FUNCTION_BLOCK "IMAC_STANDBY_CALL"
TITLE =Function calls for STANDBY objects
//*********************************************************************
//* Important : FB84 is only for use with FB80 (MOTOR1) !             *
//* STBY-Function for 2-speed or 2-direction drive is not available ! *
//*                                                                   *
//* Pumps 1 & 2 have to be allocated in different PLCs !              *
//* One PLC has the Standby Function AND one 'local' pump (MOTOR1)    *
//* The other PLCs has just one 'remote' pump (MOTOR1).               *
//* Both PLCs have to be linked by a Simatic data link to exchange    *
//* the Status & Command Words (ASTAT / ACOM) between STANDBY         *
//* function block and the 'remote' pump.                             *
//*********************************************************************
//
//Parameter Description for Function STANDBY (FB84):
//--------------------------------------------------
//OBJ:    Ascending Object number for STANDBY (1...x)
//
//C_O:    'CHANGE OVER' Input
//                      0 = Nothing to do
//                      1 = Change over command
//
//GSTA:   'GROUP START' Input
//                      0 = Nothing to do
//                      1 = Group Start (start one Motor, the other is in Standby)
//
//GSTO:   'GROUP STOP'  Input
//                      0 = Nothing to do
//                      1 = Group Start (start one Motor, the other is in Standby)
//
//FALT:   'EXT. FAULT'  Input
//                      0 = OK
//                      1 = Fault
//
//STAA:   'AUTO' Mode   Status Interface from MOTOR1 A
//                      Bit  8       : Running
//                      Bit  9       : Local
//                      Bit 10       : Manual
//                      Bit 11       : Auto
//                      Bit 12       : Failure
//                      Bit 13       : BlackOut
//                      Bit 14       : Starting
//                      Bit 15       : Restarting
//
//STAB:   'AUTO' Mode   Status Interface from MOTOR1 B (Bit assignment like STAA)
//
//PCONF:   (leave empty, refers to local instance data in Instance DB)
//
//ENAB:   'SPARE'       (not used)
//
//ACOA:   'AUTO' Mode   Command Interface to MOTOR1 A
//                      Bit  0       : BlackoutStart
//                      Bit  1       : StandbyActive
//                      Bit  7       : FetchData Command
//                      Bit  8       : Start Command
//                      Bit  9       : Stop  Command
//                      Bit 10       : Failure input from Automatic Function
//                      Bit 11       : Lock 'Start / Stop'
//                      Bit 12       : Emergency Off Command
//
//ACOB:   'AUTO' Mode   Command Interface to MOTOR1 B (Bit assignment like ACOA)
//
//OSSTAT:  OS Status Word (not used)
//
//OSALARM: OS Alarm Word  (not used)
//
//OSCOM:   OS Command Interface
//                      Bit  0       : Change Over  Command
//                      Bit  1       : Stop   Command
AUTHOR : HottendU
FAMILY : IMAC
VERSION : 0.2


VAR
  Standby_No001 : "IMAC_STANDBY";
  Standby_No002 : "IMAC_STANDBY";
  Standby_No003 : "IMAC_STANDBY";
  Standby_No004 : "IMAC_STANDBY";
  Standby_No005 : "IMAC_STANDBY";
  Standby_No006 : "IMAC_STANDBY";
  Standby_No007 : "IMAC_STANDBY";
  Standby_No008 : "IMAC_STANDBY";
  Standby_No009 : "IMAC_STANDBY";
  Standby_No010 : "IMAC_STANDBY";
END_VAR
BEGIN
NETWORK
TITLE =STANDBY Number 001

// Fetch 'ASTAT' Automatic Status Word' from first Pump ('local')
      L     "IMAC_MOTOR1_I/O".MOTOR1_005_ASTAT;
      T     "IMAC_STANDBY_I/O".STANDBY_001_STAA;

// Fetch 'ASTAT' Automatic Status Word'from Second Pump ('remote')
      L     "IMAC_MOTOR1_I/O".MOTOR1_006_ASTAT;
      T     "IMAC_STANDBY_I/O".STANDBY_001_STAB;

// Call Stanbdby Function
      CALL #Standby_No001 (
           OBJ                      := 1,
           C_O                      := E      9.2,
           GSTA                     := E      9.3,
           GSTO                     := E      9.4,
           FALT                     := E      9.5,
           STAA                     := "IMAC_STANDBY_I/O".STANDBY_001_STAA,
           STAB                     := "IMAC_STANDBY_I/O".STANDBY_001_STAB,
           ACOA                     := "IMAC_STANDBY_I/O".STANDBY_001_ACOA,
           ACOB                     := "IMAC_STANDBY_I/O".STANDBY_001_ACOB,
           OSSTAT                   := "IMAC_STANDBY_I/O".STANDBY_001_OSSTAT,
           OSALARM                  := "IMAC_STANDBY_I/O".STANDBY_001_OSALARM,
           OSCOM                    := "IMAC_STANDBY_I/O".STANDBY_001_OSCOM);

// Put 'ACOM' Automatic Command Word to first Pump (local')
      L     "IMAC_STANDBY_I/O".STANDBY_001_ACOA;
      T     "IMAC_MOTOR1_I/O".MOTOR1_005_ACOM;

// Put 'ACOM' Automatic Command Word to second Pump ('remote')
      L     "IMAC_STANDBY_I/O".STANDBY_001_ACOB;
      T     "IMAC_MOTOR1_I/O".MOTOR1_006_ACOM;
NETWORK
TITLE =STANDBY Number 002

//*********** END of function Processing ! *******************************************************************
      BEA   ; // Move this Instruction down to the next Network to add one object !
//************************************************************************************************************

      CALL #Standby_No002 (
           OBJ                      := 2,
           STAA                     := "IMAC_STANDBY_I/O".STANDBY_002_STAA,
           STAB                     := "IMAC_STANDBY_I/O".STANDBY_002_STAB,
           ACOA                     := "IMAC_STANDBY_I/O".STANDBY_002_ACOA,
           ACOB                     := "IMAC_STANDBY_I/O".STANDBY_002_ACOB,
           OSSTAT                   := "IMAC_STANDBY_I/O".STANDBY_002_OSSTAT,
           OSALARM                  := "IMAC_STANDBY_I/O".STANDBY_002_OSALARM,
           OSCOM                    := "IMAC_STANDBY_I/O".STANDBY_002_OSCOM);

NETWORK
TITLE =STANDBY Number 003

      CALL #Standby_No003 (
           OBJ                      := 3,
           STAA                     := "IMAC_STANDBY_I/O".STANDBY_003_STAA,
           STAB                     := "IMAC_STANDBY_I/O".STANDBY_003_STAB,
           ACOA                     := "IMAC_STANDBY_I/O".STANDBY_003_ACOA,
           ACOB                     := "IMAC_STANDBY_I/O".STANDBY_003_ACOB,
           OSSTAT                   := "IMAC_STANDBY_I/O".STANDBY_003_OSSTAT,
           OSALARM                  := "IMAC_STANDBY_I/O".STANDBY_003_OSALARM,
           OSCOM                    := "IMAC_STANDBY_I/O".STANDBY_003_OSCOM);

NETWORK
TITLE =STANDBY Number 004

      CALL #Standby_No004 (
           OBJ                      := 4,
           STAA                     := "IMAC_STANDBY_I/O".STANDBY_004_STAA,
           STAB                     := "IMAC_STANDBY_I/O".STANDBY_004_STAB,
           ACOA                     := "IMAC_STANDBY_I/O".STANDBY_004_ACOA,
           ACOB                     := "IMAC_STANDBY_I/O".STANDBY_004_ACOB,
           OSSTAT                   := "IMAC_STANDBY_I/O".STANDBY_004_OSSTAT,
           OSALARM                  := "IMAC_STANDBY_I/O".STANDBY_004_OSALARM,
           OSCOM                    := "IMAC_STANDBY_I/O".STANDBY_004_OSCOM);

NETWORK
TITLE =STANDBY Number 005

      CALL #Standby_No005 (
           OBJ                      := 5,
           STAA                     := "IMAC_STANDBY_I/O".STANDBY_005_STAA,
           STAB                     := "IMAC_STANDBY_I/O".STANDBY_005_STAB,
           ACOA                     := "IMAC_STANDBY_I/O".STANDBY_005_ACOA,
           ACOB                     := "IMAC_STANDBY_I/O".STANDBY_005_ACOB,
           OSSTAT                   := "IMAC_STANDBY_I/O".STANDBY_005_OSSTAT,
           OSALARM                  := "IMAC_STANDBY_I/O".STANDBY_005_OSALARM,
           OSCOM                    := "IMAC_STANDBY_I/O".STANDBY_005_OSCOM);

NETWORK
TITLE =STANDBY Number 006

      CALL #Standby_No006 (
           OBJ                      := 6,
           STAA                     := "IMAC_STANDBY_I/O".STANDBY_006_STAA,
           STAB                     := "IMAC_STANDBY_I/O".STANDBY_006_STAB,
           ACOA                     := "IMAC_STANDBY_I/O".STANDBY_006_ACOA,
           ACOB                     := "IMAC_STANDBY_I/O".STANDBY_006_ACOB,
           OSSTAT                   := "IMAC_STANDBY_I/O".STANDBY_006_OSSTAT,
           OSALARM                  := "IMAC_STANDBY_I/O".STANDBY_006_OSALARM,
           OSCOM                    := "IMAC_STANDBY_I/O".STANDBY_006_OSCOM);

NETWORK
TITLE =STANDBY Number 007

      CALL #Standby_No007 (
           OBJ                      := 7,
           STAA                     := "IMAC_STANDBY_I/O".STANDBY_007_STAA,
           STAB                     := "IMAC_STANDBY_I/O".STANDBY_007_STAB,
           ACOA                     := "IMAC_STANDBY_I/O".STANDBY_007_ACOA,
           ACOB                     := "IMAC_STANDBY_I/O".STANDBY_007_ACOB,
           OSSTAT                   := "IMAC_STANDBY_I/O".STANDBY_007_OSSTAT,
           OSALARM                  := "IMAC_STANDBY_I/O".STANDBY_007_OSALARM,
           OSCOM                    := "IMAC_STANDBY_I/O".STANDBY_007_OSCOM);

NETWORK
TITLE =STANDBY Number 008

      CALL #Standby_No008 (
           OBJ                      := 8,
           STAA                     := "IMAC_STANDBY_I/O".STANDBY_008_STAA,
           STAB                     := "IMAC_STANDBY_I/O".STANDBY_008_STAB,
           ACOA                     := "IMAC_STANDBY_I/O".STANDBY_008_ACOA,
           ACOB                     := "IMAC_STANDBY_I/O".STANDBY_008_ACOB,
           OSSTAT                   := "IMAC_STANDBY_I/O".STANDBY_008_OSSTAT,
           OSALARM                  := "IMAC_STANDBY_I/O".STANDBY_008_OSALARM,
           OSCOM                    := "IMAC_STANDBY_I/O".STANDBY_008_OSCOM);

NETWORK
TITLE =STANDBY Number 009

      CALL #Standby_No009 (
           OBJ                      := 9,
           STAA                     := "IMAC_STANDBY_I/O".STANDBY_009_STAA,
           STAB                     := "IMAC_STANDBY_I/O".STANDBY_009_STAB,
           ACOA                     := "IMAC_STANDBY_I/O".STANDBY_009_ACOA,
           ACOB                     := "IMAC_STANDBY_I/O".STANDBY_009_ACOB,
           OSSTAT                   := "IMAC_STANDBY_I/O".STANDBY_009_OSSTAT,
           OSALARM                  := "IMAC_STANDBY_I/O".STANDBY_009_OSALARM,
           OSCOM                    := "IMAC_STANDBY_I/O".STANDBY_009_OSCOM);

NETWORK
TITLE =STANDBY Number 0010

      CALL #Standby_No010 (
           OBJ                      := 10,
           STAA                     := "IMAC_STANDBY_I/O".STANDBY_010_STAA,
           STAB                     := "IMAC_STANDBY_I/O".STANDBY_010_STAB,
           ACOA                     := "IMAC_STANDBY_I/O".STANDBY_010_ACOA,
           ACOB                     := "IMAC_STANDBY_I/O".STANDBY_010_ACOB,
           OSSTAT                   := "IMAC_STANDBY_I/O".STANDBY_010_OSSTAT,
           OSALARM                  := "IMAC_STANDBY_I/O".STANDBY_010_OSALARM,
           OSCOM                    := "IMAC_STANDBY_I/O".STANDBY_010_OSCOM);

END_FUNCTION_BLOCK

